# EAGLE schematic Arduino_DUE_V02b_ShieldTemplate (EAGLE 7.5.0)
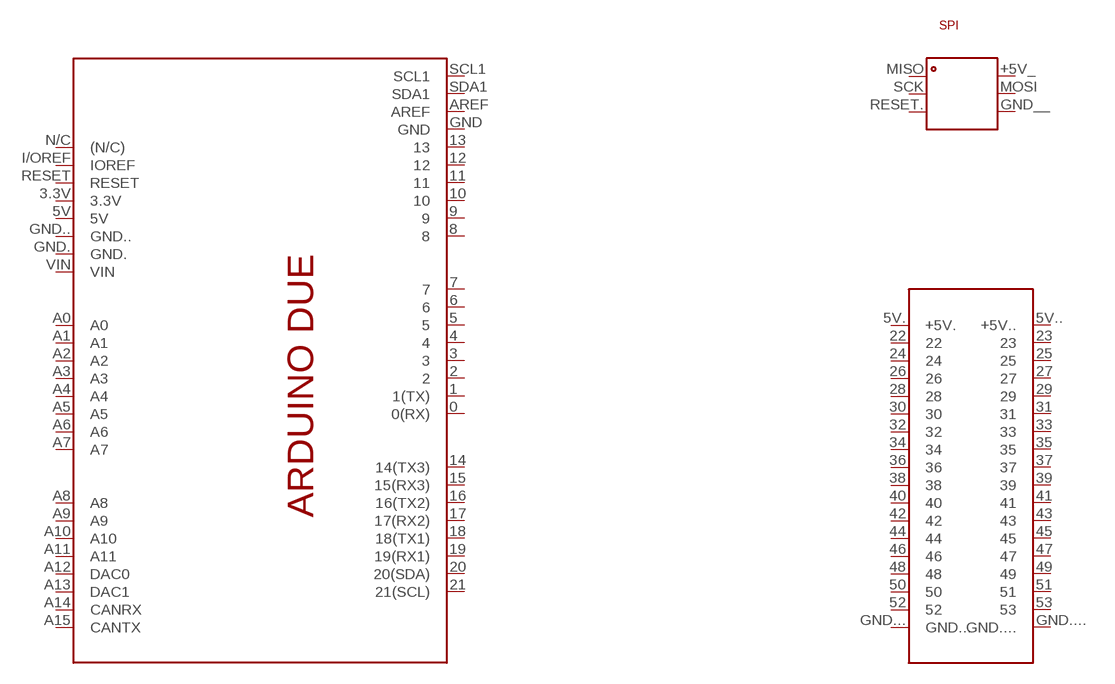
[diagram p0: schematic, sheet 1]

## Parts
PCB1  ARDUINO_DUE_REDUCED  [ARDUINO_DUE_REDUCED]
Unconnected: PCB1.0(0(RX)) PCB1.1(1(TX)) PCB1.2 PCB1.3 PCB1.3.3V PCB1.4 PCB1.5 PCB1.5V PCB1.5V.(+5V.) PCB1.5V..(+5V..) PCB1.6 PCB1.7 PCB1.8 PCB1.9 PCB1.10 PCB1.11 PCB1.12 PCB1.13 PCB1.14(14(TX3)) PCB1.15(15(RX3)) PCB1.16(16(TX2)) PCB1.17(17(RX2)) PCB1.18(18(TX1)) PCB1.19(19(RX1)) PCB1.20(20(SDA)) PCB1.21(21(SCL)) PCB1.22 PCB1.23 PCB1.24 PCB1.25 PCB1.26 PCB1.27 PCB1.28 PCB1.29 PCB1.30 PCB1.31 PCB1.32 PCB1.33 PCB1.34 PCB1.35 PCB1.36 PCB1.37 PCB1.38 PCB1.39 PCB1.40 PCB1.41 PCB1.42 PCB1.43 PCB1.44 PCB1.45 PCB1.46 PCB1.47 PCB1.48 PCB1.49 PCB1.50 PCB1.51 PCB1.52 PCB1.53 PCB1.+5V_ PCB1.A0 PCB1.A1 PCB1.A2 PCB1.A3 PCB1.A4 PCB1.A5 PCB1.A6 PCB1.A7 PCB1.A8 PCB1.A9 PCB1.A10 PCB1.A11 PCB1.A12(DAC0) PCB1.A13(DAC1) PCB1.A14(CANRX) PCB1.A15(CANTX) PCB1.AREF PCB1.GND PCB1.GND. PCB1.GND.. PCB1.GND... PCB1.GND.... PCB1.GND__ PCB1.I/OREF(IOREF) PCB1.MISO PCB1.MOSI PCB1.N/C((N/C)) PCB1.RESET PCB1.RESET. PCB1.SCK PCB1.SCL1 PCB1.SDA1 PCB1.VIN

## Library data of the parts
PCB1 = E14_Arduino_revC:ARDUINO_DUE_REDUCED: Device for representing an Arduino Due board with a footprint in an EAGLE design. Created by Dave Young for Element14. More EAGLE documentation at: http://www.element14.com/community/community/knode/cadsoft_eagle

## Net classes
0 default: width 0.203 mm, drill 0.305 mm, clearance 0.203 mm
1 USB: drill 0.406 mm, clearance 0.203 mm to class 0, clearance 0.406 mm
2 gnd: width 0.305 mm, drill 0.406 mm, clearance 0.203 mm to class 0, clearance 0.203 mm
3 usbvcc: width 0.61 mm, drill 0.508 mm, clearance 0.203 mm to class 0, clearance 0.254 mm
